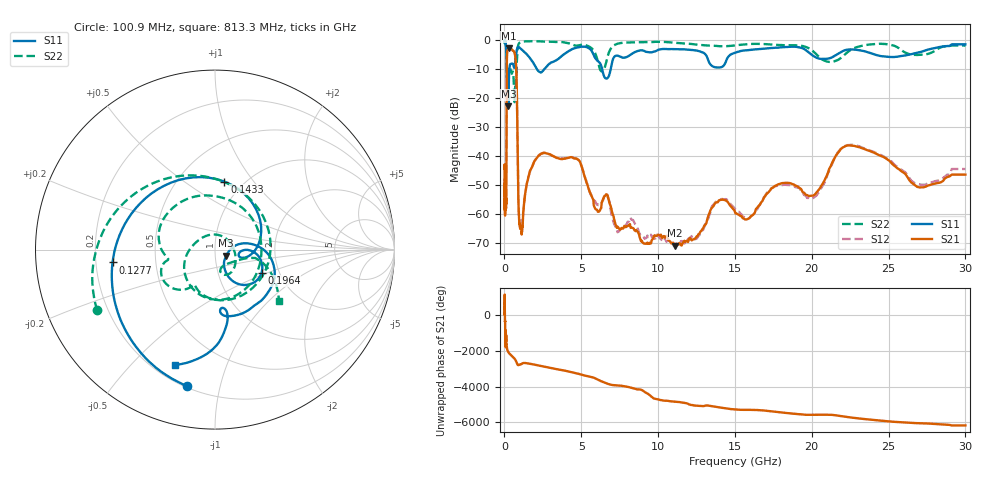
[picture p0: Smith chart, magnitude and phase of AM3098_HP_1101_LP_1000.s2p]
! Date/Time: Thu, Feb 28, 2019 8:45 AM
! Network Analyzer: Agilent Technologies E8364B Rev: A.07.50.67
! Sweep from 0.010 to 30.000 GHz, 1601 Points, Sweep Type: LOG
! Power Supply: 5.022 V, 0.002 A
# Hz S DB R 50
!freq MagS11 AngS11 MagS21 AngS21 MagS12 AngS12 MagS22 AngS22
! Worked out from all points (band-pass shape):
!   1601 points, 10 MHz to 30 GHz, reference 50 ohm
!   highest |S21| = -3.03 dB at 266.5 MHz (marker M1); lowest = -70.8 dB at 11.08 GHz (marker M2)
!   |S21| within 3 dB of the highest: 159.2 MHz to 707.4 MHz (548.2 MHz wide, 127 % of centre)
!   lowest |S11| = -22.9 dB at 252.2 MHz (marker M3), VSWR 1.15, Z = 56.5 - j3.92 ohm
!   |S11| at or under -10 dB: 148 MHz to 322.5 MHz (174.5 MHz wide, 74.2 % of centre); 2.094 GHz to 2.62 GHz (526 MHz wide, 22.3 % of centre); 6.353 GHz to 6.92 GHz (567.6 MHz wide, 8.55 % of centre)
!   |S22| runs from -21.5 to -0.5 dB; largest |S21 - S12| = 0.012
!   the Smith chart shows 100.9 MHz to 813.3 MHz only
!   S11 on the Smith chart (normalised r, x): 100.9 MHz: 0.21, -0.79; 127.7 MHz: 0.27, -0.06; 143.3 MHz: 0.82, +0.73; 196.4 MHz: 1.62, -0.46; 813.3 MHz: 0.28, -0.67
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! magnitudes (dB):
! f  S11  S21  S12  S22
! 10 MHz  -0.4  -44.4  -45.1  -0.6
! 38.04 MHz  -0.3  -58.6  -60.0  -0.8
! 100.9 MHz  -2.2  -56.5  -54.4  -2.6
! 127.7 MHz  -4.8  -41.5  -41.2  -6.2
! 143.3 MHz  -8.3  -15.9  -15.8  -10.3
! 144.7 MHz  -8.8  -14.2  -14.2  -10.4
! 196.4 MHz  -10.8  -3.8  -3.8  -9.6
! 252.2 MHz  -22.9  -3.1  -3.0  -11.5
! 266.5 MHz  -19.5  -3.0  -3.0  -11.4
! 550.5 MHz  -8.4  -3.8  -3.8  -11.1
! 655.8 MHz  -9.4  -4.5  -4.5  -21.5
! 813.3 MHz  -3.4  -20.2  -20.2  -6.8
! 907.9 MHz  -2.5  -55.7  -55.6  -1.7
! 1.004 GHz  -2.9  -64.6  -62.4  -1.0
! 2.084 GHz  -9.9  -40.8  -40.7  -0.6
! 4.734 GHz  -2.7  -41.1  -41.1  -2.1
! 6.36 GHz  -10.1  -55.6  -55.9  -11.0
! 7.926 GHz  -6.1  -64.4  -63.6  -1.0
! 11.08 GHz  -3.3  -70.8  -70.8  -1.1
! 20.1 GHz  -5.6  -53.6  -54.4  -4.1
! 22.56 GHz  -3.4  -36.4  -36.2  -3.5
! 30 GHz  -1.6  -46.4  -44.5  -2.1
